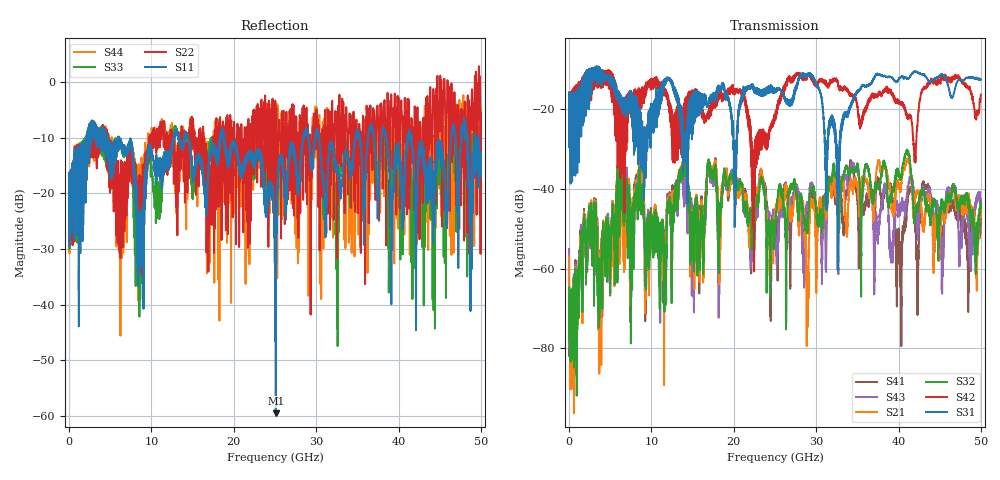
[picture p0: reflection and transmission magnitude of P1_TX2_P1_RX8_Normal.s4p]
!Keysight Technologies,N5225B,MY57041031,A.13.20.10
!Date: Friday, May 31, 2019 11:25:42
!Correction: S11(Full 4 Port(1,2,3,4))
!S12(Full 4 Port(1,2,3,4))
!S13(Full 4 Port(1,2,3,4))
!S14(Full 4 Port(1,2,3,4))
!S21(Full 4 Port(1,2,3,4))
!S22(Full 4 Port(1,2,3,4))
!S23(Full 4 Port(1,2,3,4))
!S24(Full 4 Port(1,2,3,4))
!S31(Full 4 Port(1,2,3,4))
!S32(Full 4 Port(1,2,3,4))
!S33(Full 4 Port(1,2,3,4))
!S34(Full 4 Port(1,2,3,4))
!S41(Full 4 Port(1,2,3,4))
!S42(Full 4 Port(1,2,3,4))
!S43(Full 4 Port(1,2,3,4))
!S44(Full 4 Port(1,2,3,4))
!S4P File: Measurements: <S11,S12,S13,S14>,
!<S21,S22,S23,S24>,
!<S31,S32,S33,S34>,
!<S41,S42,S43,S44>:
# Hz S  dB  R 50.0
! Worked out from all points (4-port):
!   5000 points, 10 MHz to 50 GHz, reference 50 ohm
!   strongest paths, dB at 10 MHz, 12.51 GHz, 25.01 GHz, 37.51 GHz, 50 GHz:
!     S31: -19.6, -13.0, -15.4, -11.2, -12.5
!     S42: -19.4, -24.5, -22.7, -16.3, -16.3
!     S32: -65.0, -52.8, -50.4, -39.2, -43.6
!     S21: -56.9, -47.5, -45.6, -33.0, -47.0
!     S43: -55.0, -49.9, -51.2, -51.1, -43.7
!     S41: -64.6, -44.9, -46.3, -37.6, -47.4
!   lowest |S11| = -59.5 dB at 25.1 GHz (marker M1), VSWR 1.00, Z = 49.9 + j0.0819 ohm
!   |S11| at or under -10 dB: 6.091 GHz to 12.71 GHz (6.616 GHz wide, 70.4 % of centre); 18.82 GHz to 28.43 GHz (9.604 GHz wide, 40.7 % of centre); 41.58 GHz to 46.39 GHz (4.81 GHz wide, 10.9 % of centre)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
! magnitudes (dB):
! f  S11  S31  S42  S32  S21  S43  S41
! 10 MHz  -19.8  -19.6  -19.4  -65.0  -56.9  -55.0  -64.6
! 8.36 GHz  -24.4  -22.2  -16.4  -40.4  -38.9  -40.2  -38.5
! 25.1 GHz  -59.5  -15.0  -20.7  -47.0  -44.3  -52.7  -46.2
! 28.89 GHz  -8.5  -11.8  -11.8  -48.3  -66.8  -43.6  -46.0
! 31.66 GHz  -11.9  -24.6  -13.3  -37.6  -38.5  -37.9  -37.6
! 32.64 GHz  -15.7  -37.3  -13.3  -40.9  -42.6  -54.1  -42.3
! 50 GHz  -12.7  -12.5  -16.3  -43.6  -47.0  -43.7  -47.4
